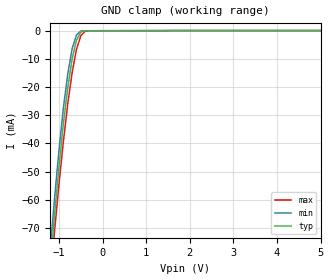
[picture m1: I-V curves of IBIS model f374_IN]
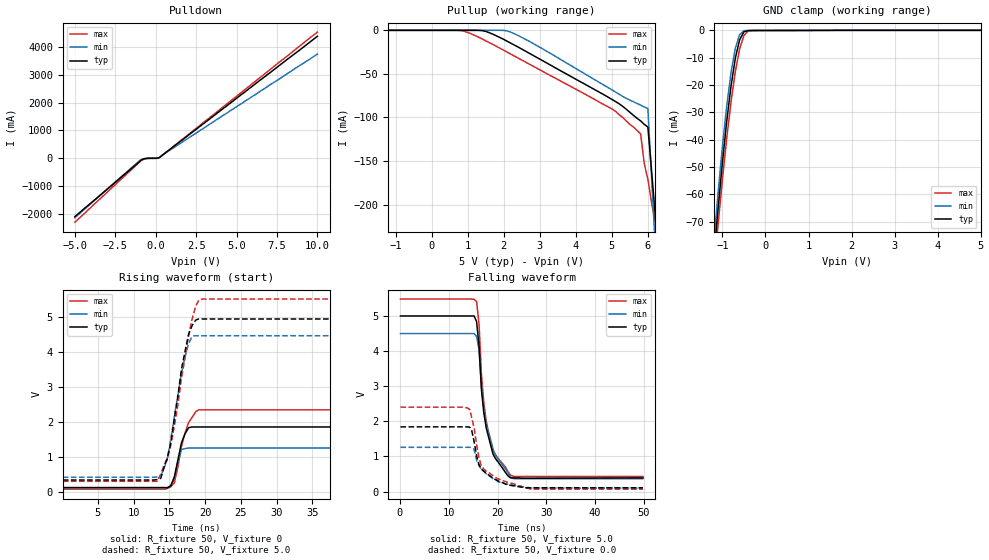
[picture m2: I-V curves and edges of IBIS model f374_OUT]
| TEXAS INSTRUMENTS INCORPORATED
| Standard Linear and Logic Group
| IBIS Model of SN74F374
| OCTAL EDGE-TRIGGERED D-TYPE FLIP-FLOPS WITH 3-STATE OUTPUTS
| SOIC 20-pin (DW), SOP 20-pin (NS), SSOP 20-pin (DB), PDIP 20-pin (N) Package
[IBIS Ver]   3.2
[Comment Char]  |_char
[File Name]   sn74f374.ibs
[File Rev]   2.1 I_die
[Date]   Nov. 05, 2000
[Source]   File originated at Texas Instruments, Inc.
[Notes]   The following is a sample IBIS file for the F374.
   - FILE REV HISTORY
   - 2.1 Re-Release IBIS file on 11/05/04
   - Power clamp data deleted as there is no power-clamp diode.
|   - All test data contained in this file are derived from
|   actual measurements.
|   - File created by Nobuhisa Ohtsubo, SLL Product Engineering.
[Disclaimer] Property of Texas Instruments Incorporated.  Unauthorized
   reproduction and/or distribution is strictly prohibited.
   This product is protected under copyright law.
   Created 2000, (C) Copyright 2000, Texas Instruments Inc.,
   All Rights Reserved.
   UNLESS THERE IS A SIGNED, WRITTEN AGREEMENT TO THE
   CONTRARY, TEXAS INSTRUMENTS () IS PROVIDING THE IBIS
   MODELS  AND WITHOUT ANY WARRANTY, EXPRESSED OR
   IMPLIED.  TI assumes no liability for:
   1) the accuracy of the IBIS models provided to your
   company;
   2) the proper functioning of these IBIS Models in your
   design or for any resulting applications; or
   3) infringement of patents, copyrights or intellectual
   property rights resulting from your use of these IBIS
   models.
   TI provides IBIS Models as a service to our customers.
   You and your company shall not distribute, sell or give
   these models to anyone else without prior written
   permission from TI.
   TI reserves the right to make changes to our products or
   to discontinue any semiconductor product or service
   without notice, and advises our customers to obtain the
   latest version of relevant information to verify, before
   placing orders, that the information being relied on is
   current.
   Please be aware that your receipt and use of the IBIS
   information provided shall serve as acceptance of these
   terms and conditions.  If you do not accept these terms,
   you should return or destroy the IBIS models and any
   other accompanying information immediately.
|   Component F374_DW
[Component]   f374_DW
[Manufacturer]  Texas Instruments, Inc.
[Package]
|   typ   min   max
R_pkg   0.038   0.033   0.045
L_pkg   5.012nH   4.110nH   6.349nH
C_pkg   0.717pF   0.530pF   0.868pF
[Pin]   signal_name   model_name   R_pin   L_pin   C_pin
1   1OE_NOT   f374_IN   0.042   6.336nH   0.865pF
2   1Q   f374_OUT   0.043   5.542nH   0.867pF
3   1D   f374_IN   0.034   4.714nH   0.732pF
4   2D   f374_IN   0.034   4.377nH   0.591pF
5   2Q   f374_OUT   0.036   4.130nH   0.533pF
6   3Q   f374_OUT   0.035   4.111nH   0.530pF
7   3D   f374_IN   0.034   4.284nH   0.583pF
8   4D   f374_IN   0.034   4.634nH   0.726pF
9   4Q   f374_OUT   0.040   5.518nH   0.865pF
10   GND   GND   0.043   6.349nH   0.866pF
11   CLK   f374_IN   0.041   6.281nH   0.861pF
12   5Q   f374_OUT   0.045   5.561nH   0.868pF
13   5D   f374_IN   0.033   4.778nH   0.742pF
14   6D   f374_IN   0.035   4.414nH   0.596pF
15   6Q   f374_OUT   0.035   4.110nH   0.533pF
16   7Q   f374_OUT   0.036   4.130nH   0.533pF
17   7D   f374_IN   0.034   4.377nH   0.591pF
18   8D   f374_IN   0.034   4.714nH   0.731pF
19   8Q   f374_OUT   0.043   5.569nH   0.868pF
20   VCC   POWER   0.042   6.308nH   0.864pF
|   Component F374_NS
[Component]   f374_NS
[Manufacturer]  Texas Instruments, Inc.
[Package]
|   typ   min   max
R_pkg   0.044   0.029   0.058
L_pkg   3.666nH   2.317nH   5.115nH
C_pkg   0.548pF   0.316pF   0.725pF
[Pin]   signal_name   model_name   R_pin   L_pin   C_pin
1   OE_NOT   f374_IN   0.058   5.115nH   0.725pF
2   1Q   f374_OUT   0.053   4.591nH   0.724pF
3   1D   f374_IN   0.049   3.754nH   0.572pF
4   2D   f374_IN   0.029   2.549nH   0.388pF
5   2Q   f374_OUT   0.031   2.317nH   0.316pF
6   3Q   f374_OUT   0.031   2.317nH   0.316pF
7   3D   f374_IN   0.029   2.556nH   0.399pF
8   4D   f374_IN   0.049   3.754nH   0.579pF
9   4Q   f374_OUT   0.053   4.591nH   0.724pF
10   GND   GND   0.058   5.115nH   0.725pF
11   CLK   f374_IN   0.058   5.115nH   0.725pF
12   5Q   f374_OUT   0.053   4.591nH   0.724pF
13   5D   f374_IN   0.049   3.754nH   0.579pF
14   6D   f374_IN   0.029   2.557nH   0.399pF
15   6Q   f374_OUT   0.031   2.317nH   0.316pF
16   7Q   f374_OUT   0.031   2.317nH   0.316pF
17   7D   f374_IN   0.029   2.557nH   0.399pF
18   8D   f374_IN   0.049   3.754nH   0.579pF
19   8Q   f374_OUT   0.053   4.591nH   0.724pF
20   VCC   POWER   0.058   5.115nH   0.725pF
|   Component F374_DB
[Component]   f374_DB
[Manufacturer]  Texas Instruments, Inc.
[Package]
|   typ   min   max
R_pkg   0.040   0.035   0.051
L_pkg   3.495nH   3.035nH   4.314nH
C_pkg   0.420pF   0.346pF   0.502pF
[Pin]   signal_name   model_name   R_pin   L_pin   C_pin
1   OE_NOT   f374_IN   0.049   4.310nH   0.502pF
2   1Q   f374_OUT   0.048   3.903nH   0.487pF
3   1D   f374_IN   0.035   3.189nH   0.396pF
4   2D   f374_IN   0.035   3.036nH   0.347pF
5   2Q   f374_OUT   0.035   3.035nH   0.367pF
6   3Q   f374_OUT   0.035   3.035nH   0.367pF
7   3D   f374_IN   0.035   3.036nH   0.347pF
8   4D   f374_IN   0.035   3.189nH   0.397pF
9   4Q   f374_OUT   0.047   3.899nH   0.488pF
10   GND   GND   0.051   4.314nH   0.500pF
11   CLK   f374_IN   0.051   4.314nH   0.500pF
12   5Q   f374_OUT   0.047   3.899nH   0.488pF
13   5D   f374_IN   0.035   3.189nH   0.397pF
14   6D   f374_IN   0.035   3.036nH   0.346pF
15   6Q   f374_OUT   0.035   3.035nH   0.367pF
16   7Q   f374_OUT   0.035   3.035nH   0.367pF
17   7D   f374_IN   0.035   3.036nH   0.346pF
18   8D   f374_IN   0.035   3.189nH   0.397pF
19   8Q   f374_OUT   0.047   3.899nH   0.488pF
20   VCC   POWER   0.051   4.314nH   0.502pF
|   Component F374_N
[Component]   f374_N
[Manufacturer]   Texas Instruments, Inc.
[Package]
|   typ   min   max
R_pkg   4.300e-02   3.800e-02   5.000e-02
L_pkg   7.384e-09   4.680e-09   1.032e-08
C_pkg   5.100e-13   2.310e-13   8.210e-13
[Pin]   signal_name   model_name   R_pin   L_pin   C_pin
1   1OE_NOT   f374_IN   4.200e-02   9.427e-09   8.100e-13
2   1Q   f374_OUT   4.600e-02   8.544e-09   4.560e-13
3   1D   f374_IN   4.800e-02   7.163e-09   4.350e-13
4   2D   f374_IN   4.000e-02   4.825e-09   2.610e-13
5   2Q   f374_OUT   4.000e-02   5.284e-09   6.480e-13
6   3Q   f374_OUT   4.000e-02   4.686e-09   2.320e-13
7   3D   f374_IN   4.000e-02   6.359e-09   4.890e-13
8   4D   f374_IN   3.800e-02   7.982e-09   4.750e-13
9   4Q   f374_OUT   4.300e-02   9.403e-09   4.750e-13
10   GND   GND   5.000e-02   1.032e-08   8.050e-13
11   CLK   f374_IN   5.000e-02   1.028e-08   8.100e-13
12   5Q   f374_OUT   4.300e-02   9.383e-09   4.770e-13
13   5D   f374_IN   3.800e-02   7.978e-09   4.760e-13
14   6D   f374_IN   4.000e-02   6.302e-09   4.920e-13
15   6Q   f374_OUT   4.000e-02   4.680e-09   2.310e-13
16   7Q   f374_OUT   4.000e-02   5.284e-09   6.480e-13
17   7D   f374_IN   4.000e-02   4.822e-09   2.610e-13
18   8D   f374_IN   4.700e-02   7.118e-09   4.390e-13
19   8Q   f374_OUT   4.600e-02   8.492e-09   4.610e-13
20   VCC   POWER   4.300e-02   9.348e-09   8.210e-13
| Models and submodels in the file (2): f374_IN (Input), f374_OUT (3-state)
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|   Model F374_IN
[Model]   f374_IN
Model_type  Input
Polarity   Inverting
Vinl = 0.8
Vinh = 2.0
| variable   typ   min   max
C_comp   1.33pf   1.00pf   1.66pf
[Temperature Range]   25   0   70
[Voltage Range]   5.0   4.75   5.25
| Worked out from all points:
|   GND clamp passes 1 mA (typ) near -0.52 V on its own axis
[GND Clamp]
|   Voltage   I(typ)   I(min)   I(max)
-5V       -1.02A     -1.07A     -940mA
-1.2V     -82.9mA    -77.6mA    -88.1mA
-1.1V     -64.9mA    -59.1mA    -70.8mA
-1V       -48.2mA    -42.3mA    -54.5mA
-900mV    -33.1mA    -27.5mA    -39.4mA
-800mV    -20.3mA    -15.4mA    -26.1mA
-700mV    -10.1mA    -6.49mA    -15mA
-600mV    -3.44mA    -1.57mA    -6.7mA
-500mV    -512uA     -145uA     -1.86mA
-400mV    -83.7uA    -69.8uA    -240uA
-300mV    -64.3uA    -65.2uA    -68.9uA
5V        19nA       36.1pA     510pA
|   Model F374_OUT
[Model]   f374_OUT
Model_type  3-state
Polarity   Non-Inverting
Enable   Active-Low
Vmeas = 1.5v
Cref = 0pf
| variable   typ   min   max
C_comp   5.8pf   4.35pf   7.25pf
[Temperature Range]   25   0   70
[Voltage Range]   5.0   4.5   5.5
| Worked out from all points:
|   slope of the pulldown table from 0 to 0.75 V, typ, clamps not added: 2.84 ohm
|   GND clamp passes 1 mA (typ) near -0.52 V on its own axis
|   rising waveform, R_fixture 50, V_fixture 0: 20-80 % time 1.16ns typ, 891ps min, 1.55ns max; typ from 0.126 V to 1.86 V
|   falling waveform, R_fixture 50, V_fixture 5.0: 20-80 % time 2.37ns typ, 2.69ns min, 2.34ns max; typ from 4.99 V to 0.391 V
|   rising waveform, R_fixture 50, V_fixture 5.0: 20-80 % time 2.16ns typ, 2ns min, 2.48ns max; typ from 0.342 V to 4.95 V
|   falling waveform, R_fixture 50, V_fixture 0.0: 20-80 % time 3.29ns typ, 4.13ns min, 3.27ns max; typ from 1.84 V to 0.109 V
[Pulldown]
|   Voltage   I(typ)   I(min)   I(max)
-5V       -2.1A      -2.14A     -2.3A
-1V       -124mA     -85mA      -139mA
-900mV    -67.6mA    -53.1mA    -85.1mA
-600mV    -11.3mA    -7.04mA    -20mA
200mV     17.1mA     11.5mA     22.1mA
500mV     149mA      147mA      144mA
10V       4.38A      3.74A      4.53A
[Pullup]
|   Voltage   II(typ)   I(min)   I(max)
-5V       649nA      17nA       2.35uA
800mV     470nA      7.21nA     -217uA
1.5V      -1.22mA    7.1nA      -12mA
2.2V      -14.8mA    -2.17mA    -27.3mA
5.6V      -97.6mA    -82mA      -111mA
5.8V      -104mA     -85.9mA    -119mA
5.9V      -108mA     -87.9mA    -153mA
6V        -111mA     -89.9mA    -171mA
6.1V      -160mA     -167mA     -197mA
6.2V      -210mA     -244mA     -220mA
6.3V      -259mA     -320mA     -244mA
10V       -2.07A     -3.16A     -1.12A
[GND Clamp]
|   Voltage   I(typ)   I(min)   I(max)
-5V       -1.02A     -1.07A     -940mA
-1.2V     -82.9mA    -77.6mA    -88.1mA
-1.1V     -64.9mA    -59.1mA    -70.8mA
-1V       -48.2mA    -42.3mA    -54.5mA
-900mV    -33.1mA    -27.5mA    -39.4mA
-800mV    -20.3mA    -15.4mA    -26.1mA
-700mV    -10.1mA    -6.49mA    -15mA
-600mV    -3.44mA    -1.57mA    -6.7mA
-500mV    -512uA     -145uA     -1.86mA
-400mV    -83.7uA    -69.8uA    -240uA
-300mV    -64.3uA    -65.2uA    -68.9uA
5V        19nA       36.2pA     518pA
[Ramp]
| variable   typ   min   max
dV/dt_r   2.064/2.212n   1.704/2.056n   2.448/2.546n
dV/dt_f   2.652/2.092n   2.364/2.401n   2.970/2.028n
R_load = 50
[Rising Waveform]
R_fixture = 50
V_fixture = 0
|   Time   V(typ)   V(min)   V(max)
97.7ps    126mV      100mV      80.1mV
14.3ns    126mV      100mV      80.1mV
15.2ns    174mV      181mV      150mV
15.7ns    432mV      400mV      262mV
16.2ns    920mV      857mV      720mV
16.7ns    1.41V      1.22V      1.31V
17.2ns    1.67V      1.24V      1.69V
17.7ns    1.84V      1.26V      1.99V
19.1ns    1.86V      1.26V      2.35V
49.8ns    1.86V      1.26V      2.35V
[Falling Waveform]
R_fixture = 50
V_fixture = 5.0
V_fixture_min = 4.5
V_fixture_max = 5.5
|   Time   V(typ)   V(min)   V(max)
97.7ps    4.99V      4.49V      5.47V
15.2ns    4.99V      4.49V      5.46V
15.7ns    4.83V      4.41V      5.4V
16.2ns    4.15V      4.04V      4.77V
16.7ns    2.89V      3V         3.33V
17.2ns    2.22V      2.36V      2.51V
17.7ns    1.8V       1.92V      1.99V
19.1ns    1.06V      1.18V      1.18V
22.6ns    395mV      423mV      477mV
49.8ns    391mV      370mV      430mV
[Rising Waveform]
R_fixture = 50
V_fixture = 5.0
V_fixture_min = 4.5
V_fixture_max = 5.5
|   Time   V(typ)   V(min)   V(max)
97.7ps    342mV      421mV      305mV
13.3ns    354mV      431mV      305mV
13.8ns    390mV      463mV      513mV
14.3ns    733mV      699mV      791mV
15.2ns    1.41V      1.5V       1.33V
16.7ns    3.52V      3.42V      3.27V
17.7ns    4.52V      4.25V      4.48V
18.7ns    4.92V      4.47V      5.33V
19.1ns    4.95V      4.47V      5.48V
49.8ns    4.95V      4.47V      5.52V
[Falling Waveform]
R_fixture = 50
V_fixture = 0.0
|   Time   V(typ)   V(min)   V(max)
97.7ps    1.84V      1.26V      2.4V
13.8ns    1.84V      1.26V      2.38V
14.3ns    1.83V      1.26V      2.33V
14.7ns    1.74V      1.24V      2.1V
15.2ns    1.42V      1.2V       1.81V
15.7ns    1.02V      900mV      1.34V
16.7ns    636mV      634mV      719mV
22.1ns    193mV      210mV      263mV
27ns      109mV      102mV      71mV
49.8ns    109mV      102mV      71mV
